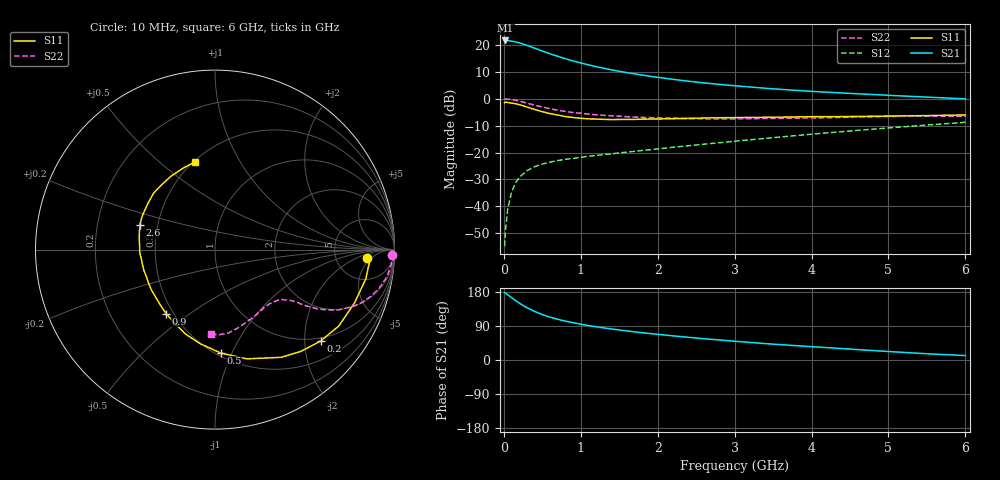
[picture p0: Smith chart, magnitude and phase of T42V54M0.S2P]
! Infineon Technologies  Discrete & RF Semiconductors
! BFR182T
! Si NPN RF Bipolar Junction Transistor in SC75
! VCE = 2.5 V  IC = 4 mA
! Common Emitter S-Parameters:  October  1999
# GHz  S  MA  R  50
!  f  S11  S21  S12  S22
! GHz  MAG  ANG  MAG  ANG  MAG  ANG  MAG  ANG
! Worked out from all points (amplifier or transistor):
!   36 points, 10 MHz to 6 GHz, reference 50 ohm
!   highest |S21| = 21.7 dB at 20 MHz (marker M1)
!   |S21| within 3 dB of that: start of sweep to 412.1 MHz
!   unconditionally stable (mu >= 1): 1.536 GHz to 4.078 GHz
!   at 250 MHz: K = 0.24, MSG = 24.2 dB, |S12| = -28.0 dB
!   at 1.4 GHz: K = 0.97, MSG = 15.7 dB, |S12| = -20.5 dB
!   at 6 GHz: K = 0.84, MSG = 4.4 dB, |S12| = -8.8 dB
!   S11 on the Smith chart (normalised r, x): 10 MHz: 11, -4; 200 MHz: 0.92, -2.37; 500 MHz: 0.53, -0.91; 900 MHz: 0.46, -0.41; 2.6 GHz: 0.40, +0.13; 6 GHz: 0.51, +0.66
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0.01  0.8497 -3.2  12.19 177.7  0.0018 68.3  0.9848 -1.7
0.02  0.8668 -3.1  12.23 177.0  0.0034 95.6  0.9922 -1.9
0.05  0.856 -10.9  12.16 172.1  0.0088 87.5  0.9854 -4.6
0.1  0.8321 -20.9  11.86 164.7  0.0181 79.5  0.9699 -9.0
0.15  0.8104 -31.7  11.52 157.1  0.0267 74.6  0.9405 -13.1
0.2  0.7781 -40.9  11.04 150.3  0.0342 71.3  0.9081 -16.6
0.25  0.7422 -49.8  10.47 143.9  0.0397 65.4  0.8707 -19.7
0.3  0.704 -58.5  9.89 138.1  0.0459 62.7  0.8342 -22.3
0.4  0.6338 -73.8  8.788 128.0  0.0544 57.0  0.7621 -26.2
0.5  0.5772 -86.8  7.771 120.0  0.061 53.7  0.7034 -28.5
0.6  0.5309 -98.9  6.901 113.1  0.0661 51.9  0.6538 -30.2
0.7  0.4986 -109.2  6.2 107.5  0.0707 50.3  0.6139 -31.2
0.9  0.449 -127.3  5.077 98.4  0.0774 49.4  0.5556 -32.5
1.1  0.4229 -142.1  4.297 90.8  0.0851 50.1  0.5194 -33.5
1.3  0.414 -154.0  3.719 84.7  0.0918 50.9  0.4921 -34.8
1.6  0.4129 -168.9  3.076 76.7  0.1017 52.6  0.4647 -36.6
2.2  0.4266 171.7  2.307 63.7  0.1251 56.7  0.4361 -42.5
2.6  0.4393 162.1  1.984 56.2  0.1428 58.7  0.4252 -47.3
3.5  0.4542 145.0  1.534 41.8  0.1889 60.3  0.4314 -59.1
4.5  0.4678 129.6  1.262 28.8  0.2519 58.8  0.4544 -73.6
5.5  0.4871 111.6  1.076 16.5  0.3253 54.6  0.4746 -86.9
6  0.5012 103.0  0.999 11.7  0.365 51.3  0.4724 -92.7
